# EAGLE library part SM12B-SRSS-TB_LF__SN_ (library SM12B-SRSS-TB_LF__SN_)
Connector Header Surface Mount, Right Angle 12 position 0.039" (1.00mm) Source: Datasheet
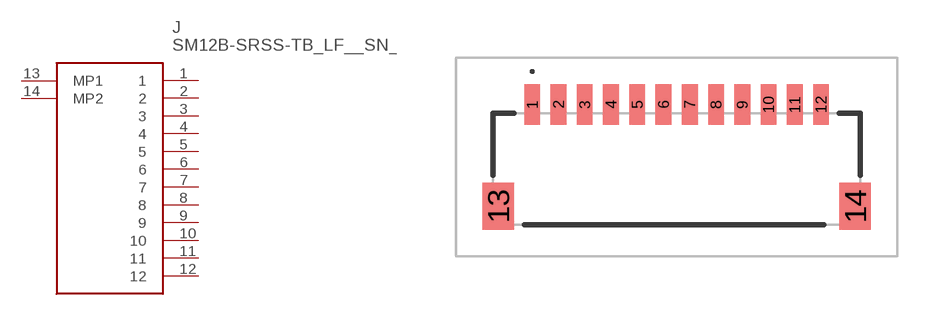
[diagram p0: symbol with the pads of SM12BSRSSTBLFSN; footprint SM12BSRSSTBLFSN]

Designator prefix J

## SM12B-SRSS-TB_LF__SN_ (Arrow_Part_Number: SM12B-SRSS-TB(LF)(SN); Arrow_Price-Stock: https://www.arrow.com/en/products/sm12b-srss-tb-lf-sn/jst-manufacturing?utm_currency=USD&region=europe; Description: Connector Header Surface Mount, Right Angle 12 position 0.039" (1.00mm); Height: 2.95mm; Manufacturer_Name: JST (JAPAN SOLDERLESS TERMINALS); Manufacturer_Part_Number: SM12B-SRSS-TB(LF)(SN); Mouser_Part_Number: N/A; Mouser_Price-Stock: https://www.mouser.co.uk/ProductDetail/JST-Commercial/SM12B-SRSS-TBLFSN?qs=QpmGXVUTftGbMQGOEOOssg%3D%3D)  [SM12BSRSSTBLFSN]
1  1
2  2
3  3
4  4
5  5
6  6
7  7
8  8
9  9
10  10
11  11
12  12
13  MP1
14  MP2

## Footprint SM12BSRSSTBLFSN (pad centres in mm)
SM12B-SRSS-TB(LF)(SN)-2
smd 0.6 x 1.55: 1 -5.5,2.287; 2 -4.5,2.287; 3 -3.5,2.287; 4 -2.5,2.287; 5 -1.5,2.287; 6 -0.5,2.287; 7 0.5,2.287; 8 1.5,2.287; 9 2.5,2.287; 10 3.5,2.287; 11 4.5,2.287; 12 5.5,2.287
smd 1.2 x 1.8: 13 -6.8,-1.588; 14 6.8,-1.588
